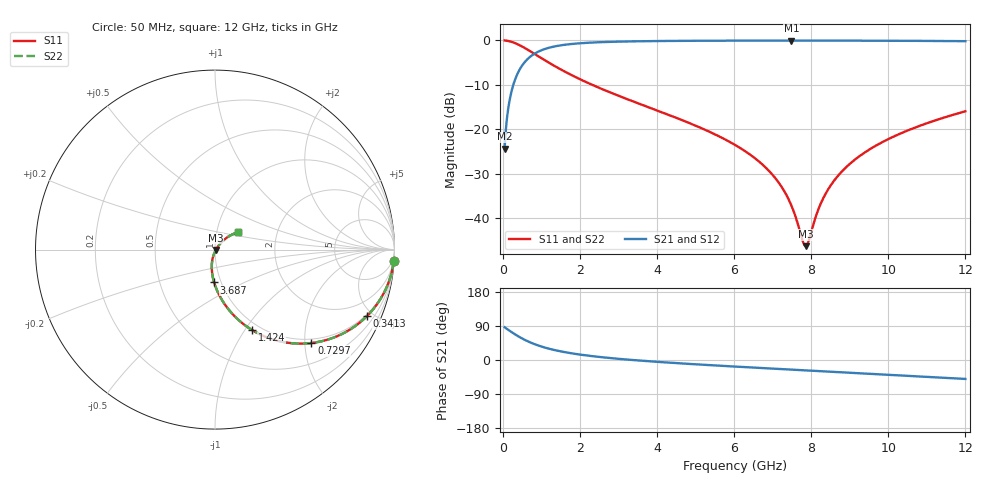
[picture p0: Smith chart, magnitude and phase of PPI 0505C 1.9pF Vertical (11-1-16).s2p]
# MHz S MA R 50
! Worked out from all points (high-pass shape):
!   1601 points, 50 MHz to 12 GHz, reference 50 ohm
!   highest |S21| = -0.05 dB at 7.489 GHz (marker M1); lowest = -24.4 dB at 50 MHz (marker M2)
!   |S21| within 3 dB of the highest: 816.8 MHz to end of sweep
!   lowest |S11| = -46.3 dB at 7.855 GHz (marker M3), VSWR 1.01, Z = 50.4 - j0.236 ohm
!   |S11| at or under -10 dB: 2.322 GHz to end of sweep
!   |S22| runs from -46.3 to 0.0 dB; largest |S21 - S12| = 0
!   S11 on the Smith chart (normalised r, x): 50 MHz: 1, -31; 341.3 MHz: 0.91, -4.61; 729.7 MHz: 0.91, -2.14; 1.424 GHz: 0.91, -1.08; 3.687 GHz: 0.93, -0.35; 12 GHz: 1.26, +0.25
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50  0.9982 -3.6  0.06028 86.4  0.06028 86.4  0.9982 -3.6
184.4375  0.976 -13.2  0.2175 76.8  0.2175 76.8  0.976 -13.2
341.2812  0.9241 -23.6  0.3814 66.3  0.3814 66.3  0.9241 -23.6
513.0625  0.8489 -33.7  0.5276 56.3  0.5276 56.3  0.8489 -33.7
729.6562  0.7476 -44.1  0.6628 45.8  0.6628 45.8  0.7476 -44.1
1058.281  0.6105 -56.0  0.7903 33.9  0.7903 33.9  0.6105 -56.0
1424.25  0.4929 -65.3  0.8679 24.5  0.8679 24.5  0.4929 -65.3
2044.156  0.3589 -75.8  0.9308 13.8  0.9308 13.8  0.3589 -75.8
3687.281  0.1833 -91.5  0.9796 -2.5  0.9796 -2.5  0.1833 -91.5
4038.312  0.1605 -93.8  0.9834 -5.0  0.9834 -5.0  0.1605 -93.8
6025  0.06671 -103.8  0.9933 -17.3  0.9933 -17.3  0.06671 -103.8
6936.188  0.03295 -104.6  0.9946 -22.4  0.9946 -22.4  0.03295 -104.6
7249.875  0.02193 -102.0  0.9947 -24.1  0.9947 -24.1  0.02193 -102.0
7488.875  0.01382 -95.6  0.9948 -25.4  0.9948 -25.4  0.01382 -95.6
7780.156  0.00554 -56.8  0.9947 -27.0  0.9947 -27.0  0.00554 -56.8
7854.844  0.004837 -29.0  0.9947 -27.4  0.9947 -27.4  0.004837 -29.0
8019.156  0.007463 20.7  0.9946 -28.2  0.9946 -28.2  0.007463 20.7
8302.969  0.01639 42.4  0.9943 -29.8  0.9943 -29.8  0.01639 42.4
8691.344  0.02978 48.1  0.9938 -31.8  0.9938 -31.8  0.02978 48.1
9251.5  0.04975 48.9  0.9928 -34.8  0.9928 -34.8  0.04975 48.9
10013.31  0.07796 46.8  0.9906 -39.0  0.9906 -39.0  0.07796 46.8
12000  0.1594 37.5  0.9797 -50.0  0.9797 -50.0  0.1594 37.5
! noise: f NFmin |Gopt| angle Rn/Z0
50  0.0008805  0.9511  1.706  0.004048
1372  0.005663  0.7605  6.166  0.004779
2701  0.008933  0.7095  10.55  0.006002
4031  0.01182  0.6795  14.97  0.007013
5360  0.01453  0.6598  19.35  0.007943
6682  0.01716  0.6469  23.64  0.008849
8012  0.01981  0.639  27.86  0.009783
9341  0.0225  0.6351  31.98  0.01077
1.067e+04  0.02529  0.6347  35.98  0.01185
1.2e+04  0.02823  0.6373  39.87  0.01305
